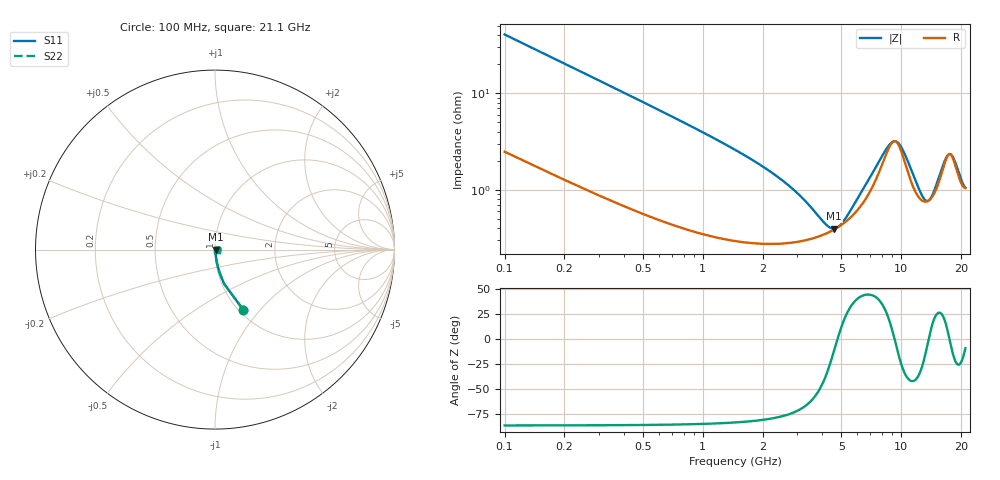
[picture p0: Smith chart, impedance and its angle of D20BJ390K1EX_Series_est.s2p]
! Dielectric Laboratories - Cap Cad
! 2777 Route 20 East
! Cazenovia, NY 13035
! Phone: (315) 655-8710
! The data contained within this file is representative of modeled device performance.
! Device performance will vary slightly from manufacturing lot to manufacturing lot.
! This performance shall not be construed as a specification nor a guarantee of performance.
! 5/31/2017 12:30:34 PM
! Part Number: D20BT390F1PX
! Temperature: 25 (°C)
# GHZ S DB R 50
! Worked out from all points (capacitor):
!   211 points, 100 MHz to 21.1 GHz, reference 50 ohm
!   read as one part in series: C = 39.1 pF near 200 MHz
!   lowest |Z| = 393 mohm at 4.6 GHz (marker M1)
!   series resonance near 4.775 GHz, so ESL is about 28 pH
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0.1  -8.65 -64.9  -0.85 21.6  -0.85 21.6  -8.65 -64.9
0.2  -14.11 -75.1  -0.28 11.3  -0.28 11.3  -14.11 -75.1
0.4  -19.99 -80.5  -0.10 5.7  -0.10 5.7  -19.99 -80.5
0.6  -23.54 -82.1  -0.06 3.8  -0.06 3.8  -23.54 -82.1
0.9  -27.18 -82.7  -0.04 2.5  -0.04 2.5  -27.18 -82.7
1.7  -33.39 -81.3  -0.03 1.2  -0.03 1.2  -33.39 -81.3
3.6  -44.21 -59.3  -0.03 0.3  -0.03 0.3  -44.21 -59.3
4.2  -47.36 -35.1  -0.03 0.1  -0.03 0.1  -47.36 -35.1
4.6  -48.14 -10.8  -0.03 0.0  -0.03 0.0  -48.14 -10.8
5.1  -46.72 16.9  -0.04 -0.1  -0.04 -0.1  -46.72 16.9
7.1  -36.96 43.7  -0.09 -0.6  -0.09 -0.6  -36.96 43.7
8.4  -31.86 26.7  -0.20 -0.7  -0.20 -0.7  -31.86 26.7
9.1  -30.31 6.0  -0.27 -0.2  -0.27 -0.2  -30.31 6.0
9.7  -30.61 -14.8  -0.25 0.4  -0.25 0.4  -30.61 -14.8
10.6  -33.44 -36.1  -0.15 0.7  -0.15 0.7  -33.44 -36.1
12.9  -41.65 -24.1  -0.07 0.2  -0.07 0.2  -41.65 -24.1
13.5  -42.44 -7.8  -0.07 0.1  -0.07 0.1  -42.44 -7.8
14.1  -41.86 8.7  -0.07 -0.1  -0.07 -0.1  -41.86 8.7
16.6  -34.17 18.5  -0.16 -0.4  -0.16 -0.4  -34.17 18.5
17.6  -32.81 -1.2  -0.20 0.0  -0.20 0.0  -32.81 -1.2
18.4  -33.69 -16.8  -0.17 0.3  -0.17 0.3  -33.69 -16.8
21.1  -39.68 -9.0  -0.09 0.1  -0.09 0.1  -39.68 -9.0
